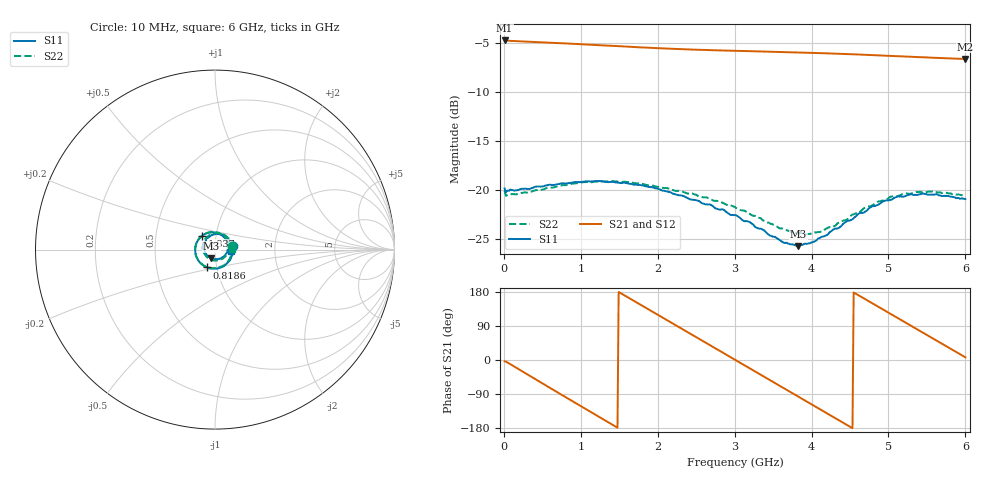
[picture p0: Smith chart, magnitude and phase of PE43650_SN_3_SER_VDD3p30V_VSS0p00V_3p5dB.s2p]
!Keysight Technologies,N5245B,MY57181451,A.13.50.07
!Date: Tuesday, May 07, 2019 07:59:51
!Correction: S11(Full 2 Port(1,2))
!S21(Full 2 Port(1,2))
!S12(Full 2 Port(1,2))
!S22(Full 2 Port(1,2))
!S2P File: Measurements: S11, S21, S12, S22:
# Hz S  dB  R 50
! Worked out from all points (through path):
!   401 points, 10 MHz to 6 GHz, reference 50 ohm
!   highest |S21| = -4.75 dB at 10 MHz (marker M1); lowest = -6.6 dB at 6 GHz (marker M2)
!   group delay of S21, straight-line fit = 329 ps
!   lowest |S11| = -25.7 dB at 3.829 GHz (marker M3), VSWR 1.11, Z = 47.8 - j4.61 ohm
!   |S11| at or under -10 dB: start of sweep to end of sweep
!   |S22| runs from -24.5 to -19.1 dB; largest |S21 - S12| = 0.0041
!   S11 on the Smith chart (normalised r, x): 10 MHz: 1.22, +0.05; 818.6 MHz: 0.90, -0.18; 1.837 GHz: 0.86, +0.14; 6 GHz: 1.20, -0.02
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1e7  -19.80 10.7  -4.75 -3.3  -4.79 -3.3  -20.04 12.3
2.1965e8  -19.87 -32.4  -4.85 -27.5  -4.90 -27.4  -20.29 -32.0
4.5925e8  -19.62 -66.2  -4.93 -56.5  -4.99 -56.5  -19.98 -65.6
8.1865e8  -19.29 -113.6  -5.06 -99.9  -5.11 -99.9  -19.44 -112.7
1.013325e9  -19.15 -138.2  -5.15 -123.3  -5.19 -123.3  -19.20 -136.5
1.432625e9  -19.17 174.0  -5.31 -173.3  -5.37 -173.3  -19.08 177.2
1.83695e9  -19.57 131.9  -5.47 138.7  -5.53 138.6  -19.43 136.2
2.01665e9  -19.89 114.1  -5.54 117.4  -5.59 117.4  -19.67 119.0
2.241275e9  -20.45 92.0  -5.62 90.9  -5.67 90.9  -20.05 97.5
2.4659e9  -20.97 69.2  -5.68 64.4  -5.73 64.5  -20.38 75.7
2.750425e9  -21.84 40.6  -5.75 30.9  -5.80 31.0  -21.07 46.9
3.005e9  -22.52 10.8  -5.80 0.9  -5.86 1.0  -21.71 19.2
3.469225e9  -24.63 -51.8  -5.90 -54.0  -5.95 -53.9  -23.41 -41.5
3.828625e9  -25.69 -112.4  -5.98 -96.5  -6.02 -96.4  -24.37 -97.4
4.008325e9  -25.29 -144.3  -6.01 -117.8  -6.06 -117.8  -24.35 -128.2
4.2629e9  -24.13 173.7  -6.08 -148.0  -6.13 -147.9  -23.77 -169.6
4.5025e9  -23.06 139.2  -6.15 -176.4  -6.20 -176.3  -22.66 154.0
4.7421e9  -21.86 108.0  -6.23 155.2  -6.28 155.4  -21.64 123.2
5.01165e9  -21.01 78.2  -6.32 123.4  -6.37 123.6  -20.73 91.2
5.4609e9  -20.34 34.9  -6.47 70.5  -6.51 70.6  -20.22 46.6
5.745425e9  -20.59 12.4  -6.56 37.0  -6.61 37.1  -20.24 22.0
6e9  -20.89 -4.7  -6.64 7.1  -6.69 7.2  -20.61 3.1
